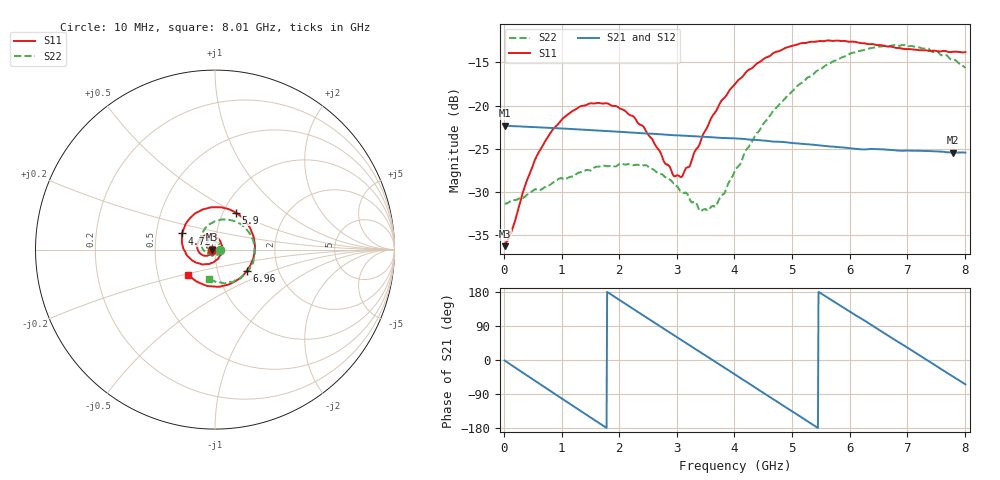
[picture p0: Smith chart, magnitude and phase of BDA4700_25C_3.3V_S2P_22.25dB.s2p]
!Agilent Technologies,E5071B,MY42404982,A.09.10
!Date: Mon Oct 20 18:12:24 2025
!Data & Calibration Information:
!Freq	S11:SOLT2(ON)	S21:SOLT2(ON)	S12:SOLT2(ON)	S22:SOLT2(ON)
# Hz S RI R 50
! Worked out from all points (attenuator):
!   801 points, 10 MHz to 8.01 GHz, reference 50 ohm
!   highest |S21| = -22.32 dB at 20 MHz (marker M1); lowest = -25.5 dB at 7.8 GHz (marker M2)
!   lowest |S11| = -36.3 dB at 10 MHz (marker M3), VSWR 1.03, Z = 48.5 - j0.115 ohm
!   |S11| at or under -10 dB: start of sweep to end of sweep
!   |S22| runs from -32.3 to -13.0 dB; largest |S21 - S12| = 0.0009
!   S11 on the Smith chart (normalised r, x): 10 MHz: 0.97, -0.00; 4.72 GHz: 0.68, +0.13; 5.9 GHz: 1.14, +0.50; 6.96 GHz: 1.38, -0.34; 8.01 GHz: 0.72, -0.21
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1e7  -0.0153 -0.00118  0.0765 -0.00168  0.0766 -0.0017  0.0271 -0.000804
2e7  -0.0156 -0.00187  0.0765 -0.00288  0.0764 -0.00316  0.027 -0.0011
6e8  -0.0411 -0.034  0.0361 -0.0655  0.036 -0.0655  0.0131 -0.0297
1.01e9  -0.0799 -0.0242  -0.0158 -0.0718  -0.0158 -0.0718  -0.0155 -0.0345
1.35e9  -0.0992 0.00865  -0.0526 -0.0499  -0.0526 -0.05  -0.0369 -0.018
2.08e9  -0.0476 0.0813  -0.0613 0.0341  -0.0614 0.0341  -0.0298 0.0346
2.68e9  0.029 0.0476  -0.00218 0.0682  -0.00228 0.0682  0.014 0.0381
2.94e9  0.0385 0.00821  0.0269 0.0617  0.027 0.0616  0.0262 0.0239
3.08e9  0.0356 -0.0148  0.0408 0.0532  0.0402 0.0534  0.0289 0.0127
3.41e9  0.00222 -0.0614  0.0619 0.0232  0.0619 0.0232  0.0212 -0.0123
3.54e9  -0.0186 -0.074  0.0651 0.00889  0.0652 0.00883  0.0137 -0.0208
3.69e9  -0.048 -0.0809  0.0647 -0.00773  0.0648 -0.00791  0.000881 -0.0265
4.01e9  -0.1152 -0.0669  0.0506 -0.0399  0.0507 -0.0398  -0.0322 -0.0265
4.72e9  -0.1835 0.0901  -0.0191 -0.0587  -0.0187 -0.0588  -0.0805 0.0534
5.35e9  -0.0603 0.2258  -0.0584 -0.0108  -0.0582 -0.0111  -0.0157 0.1485
5.9e9  0.1156 0.2063  -0.042 0.0387  -0.0421 0.0384  0.1087 0.1579
6.35e9  0.2089 0.0875  -0.00515 0.0557  -0.0051 0.0554  0.1969 0.0839
6.68e9  0.2177 -0.028  0.025 0.0495  0.0251 0.0494  0.2206 -0.00161
6.96e9  0.1767 -0.1175  0.0439 0.0329  0.0439 0.0325  0.2093 -0.078
7.42e9  0.0397 -0.203  0.0539 -0.00712  0.054 -0.00724  0.1214 -0.1666
7.8e9  -0.0914 -0.1834  0.0384 -0.0369  0.0383 -0.037  0.0172 -0.1833
8.01e9  -0.1482 -0.1402  0.0231 -0.0481  0.0233 -0.0481  -0.0328 -0.1622
